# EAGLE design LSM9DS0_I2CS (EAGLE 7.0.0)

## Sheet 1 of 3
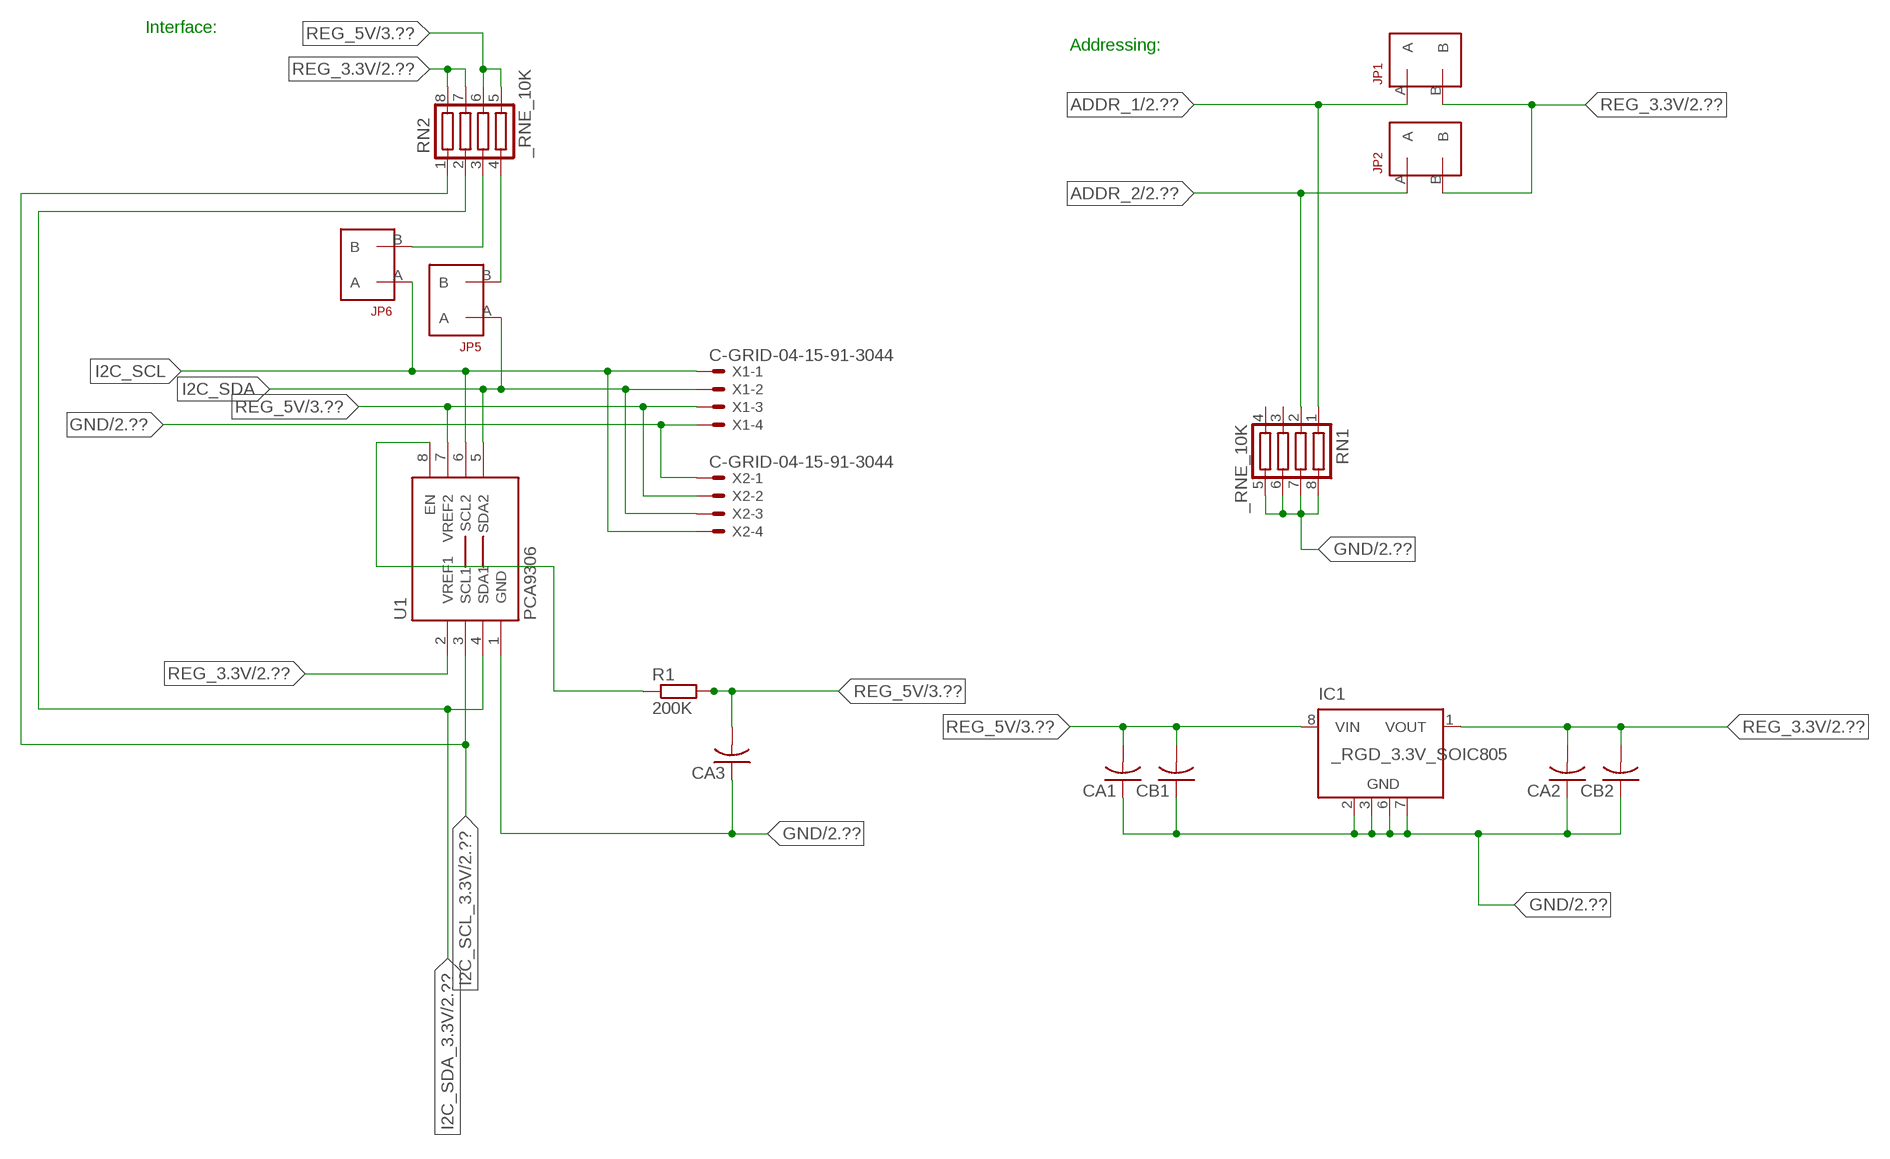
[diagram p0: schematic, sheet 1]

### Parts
CA1  CC1206KRX7R9BB104  [.1UF]
CA2  CC1206KRX7R9BB104  [.1UF]
CA3  CC1206KRX7R9BB104  [.1UF]
CB1  TMK316F106ZL-TC1206K  [TMK316F106ZL-T]
CB2  TMK316F106ZL-TC1206K  [TMK316F106ZL-T]
IC1  _RGD_3.3V_SOIC805  [_RGC_3.3V_SOIC8]
JP1  JUMPER_1X2_2MM  [JUMPER_1X2_2MM]
JP2  JUMPER_1X2_2MM  [JUMPER_1X2_2MM]
JP5  JUMPER_1X2_2MM  [JUMPER_1X2_2MM]
JP6  JUMPER_1X2_2MM  [JUMPER_1X2_2MM]
R1  200K  RESISTOR_SMT-0603  [R603]
RN1  _RNE_10K  [RNE]
RN2  _RNE_10K  [RNE]
U1  PCA9306  PCA9306_NCD  [PSOP-8]
X1  C-GRID-04-15-91-3044  [15-91-04]
X2  C-GRID-04-15-91-3044  [15-91-04]

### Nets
ADDR_1: JP1.A RN1.1 ; also sheet 2
ADDR_2: JP2.A RN1.2 ; also sheet 2
GND: CA1.1 CA2.1 CA3.1 CB1.1 CB2.1 IC1.2(GND) IC1.3(GND) IC1.6(GND) IC1.7(GND) RN1.5 RN1.6 RN1.7 RN1.8 U1.1(GND) X1.4 X2.1 ; also sheet 2,3
I2C_SCL: JP6.A U1.6(SCL2) X1.1 X2.4
I2C_SCL_3.3V: RN2.1 U1.3(SCL1) ; also sheet 2
I2C_SDA: JP5.A U1.5(SDA2) X1.2 X2.3
I2C_SDA_3.3V: RN2.2 U1.4(SDA1) ; also sheet 2
N$1: JP6.B RN2.3
N$2: JP5.B RN2.4
N$3: R1.1 U1.8(EN)
REG_3.3V: CA2.2 CB2.2 IC1.1(VOUT) JP1.B JP2.B RN2.7 RN2.8 U1.2(VREF1) ; also sheet 2
REG_5V: CA1.2 CA3.2 CB1.2 IC1.8(VIN) R1.2 RN2.5 RN2.6 U1.7(VREF2) X1.3 X2.2 ; also sheet 3
Unconnected: IC1.4(NC) IC1.5(NC) RN1.3 RN1.4

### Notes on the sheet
- Interface:
- Addressing:

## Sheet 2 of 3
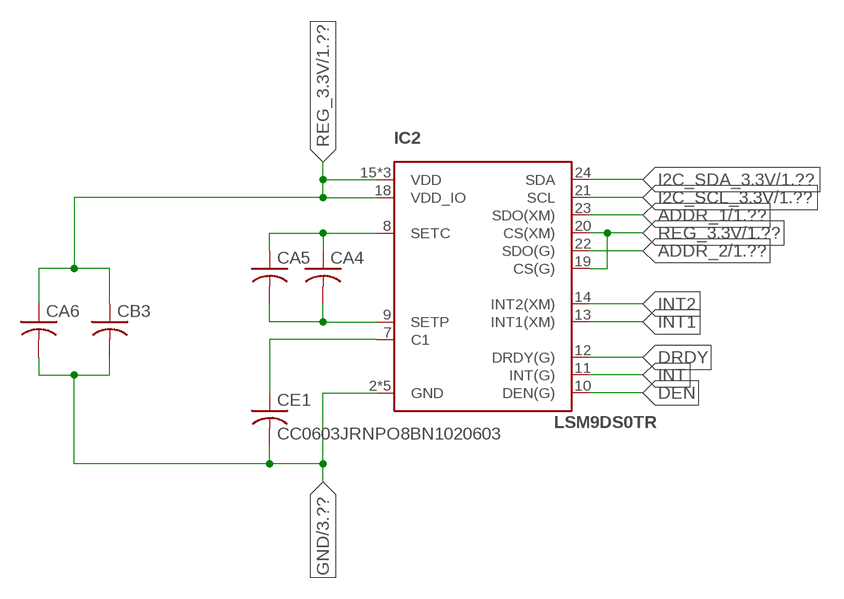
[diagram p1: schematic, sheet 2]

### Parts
CA4  CC1206KRX7R9BB104  [.1UF]
CA5  CC1206KRX7R9BB104  [.1UF]
CA6  CC1206KRX7R9BB104  [.1UF]
CB3  TMK316F106ZL-TC1206K  [TMK316F106ZL-T]
CE1  CC0603JRNPO8BN1020603  [CC0603JRNPO8BN102]
IC2  LSM9DS0TR  LSM9DS0  [LGA-24]

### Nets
ADDR_1: IC2.23(SDO(XM)) ; also sheet 1
ADDR_2: IC2.22(SDO(G)) ; also sheet 1
DEN: IC2.10(DEN(G))
DRDY: IC2.12(DRDY(G))
GND: CA6.2 CB3.2 CE1.2 IC2.2(GND) IC2.3(GND) IC2.4(GND) IC2.5(GND) IC2.6(GND) ; also sheet 1,3
I2C_SCL_3.3V: IC2.21(SCL) ; also sheet 1
I2C_SDA_3.3V: IC2.24(SDA) ; also sheet 1
INT: IC2.11(INT(G))
INT1: IC2.13(INT1(XM))
INT2: IC2.14(INT2(XM))
N$17: CA4.2 CA5.2 IC2.9(SETP)
N$18: CE1.1 IC2.7(C1)
N$19: CA4.1 CA5.1 IC2.8(SETC)
REG_3.3V: CA6.1 CB3.1 IC2.15(VDD) IC2.16(VDD) IC2.17(VDD) IC2.18(VDD_IO) IC2.19(CS(G)) IC2.20(CS(XM)) ; also sheet 1

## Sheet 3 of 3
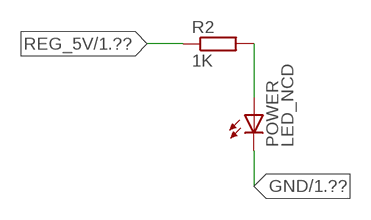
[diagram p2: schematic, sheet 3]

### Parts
POWER  LED_NCD  [CHIPLED_0603]
R2  1K  RESISTOR_SMT-0402  [R402]

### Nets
GND: POWER.C ; also sheet 1,2
N$4: POWER.A R2.2
REG_5V: R2.1 ; also sheet 1

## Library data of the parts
CA1-CA3 = NCD_ULTIMATE_LIBRARY:CC1206KRX7R9BB104: Capacitor CA .1uF 50V SMT C1206K CC1206KRX7R9BB104
CA4-CA6 = NCD_ULTIMATE_LIBRARY (2):CC1206KRX7R9BB104: Capacitor CA .1uF 50V SMT C1206K CC1206KRX7R9BB104
CB1 CB2 = NCD_ULTIMATE_LIBRARY:TMK316F106ZL-T: Capacitor CB 10uF SMT 1206 TMK316F106ZL-T
CB3 = NCD_ULTIMATE_LIBRARY (2):TMK316F106ZL-T: Capacitor CB 10uF SMT 1206 TMK316F106ZL-T
CE1 = NCD_ULTIMATE_LIBRARY (2):CC0603JRNPO8BN102: Capacitor CE 1uF SMT CC0603JRNPO8BN102 0603
IC1 = NCD_ULTIMATE_LIBRARY:_RGD_3.3V_SOIC8: Regulator Linear 3.3V Chip Positive VOLTAGE REGULATOR Digikey 497-1199-2-ND/L78L33ACD13TR
IC2 = NCD_ULTIMATE_KAMNA:LSM9DS0
JP1 JP2 JP5 JP6 = NCD_ULTIMATE_CONNECTORS:JUMPER_1X2_2MM
POWER = NCD_ULTIMATE_LIBRARY:LED_NCD: LED Digikey 754-1132-2-ND/APT2012SRCPRV
R1 R2 = NCD_ULTIMATE_LIBRARY:RESISTOR_SMT: NCD Resistor
RN1 RN2 = NCD_ULTIMATE_LIBRARY:_RNE_10K: Resistor Array RNE SMT 10K x 4 Single Resistor Source: http://www.ctscorp.com/components/Datasheets/CTSChipArrayDs.pdf Digikey 742C083103JPTR-ND/742C083103JP; OC_FARNELL: unknown; OC_NEWARK: unknown
U1 = NCD_ULTIMATE_LIBRARY:PCA9306_NCD: NCD Bidirectional I2C level shifter. NOT compatible with all available part number pinout schemes- DOUBLE CHECK!!!; PROD_ID: IC-10023
X1 X2 = NCD_ULTIMATE_CONNECTORS:C-GRID-04: CONNECTOR 4-Pos I2C wire to board 2.54 mm (0.100") pitch header Digikey WM1342-ND/0015912045; OC_FARNELL: unknown; OC_NEWARK: unknown

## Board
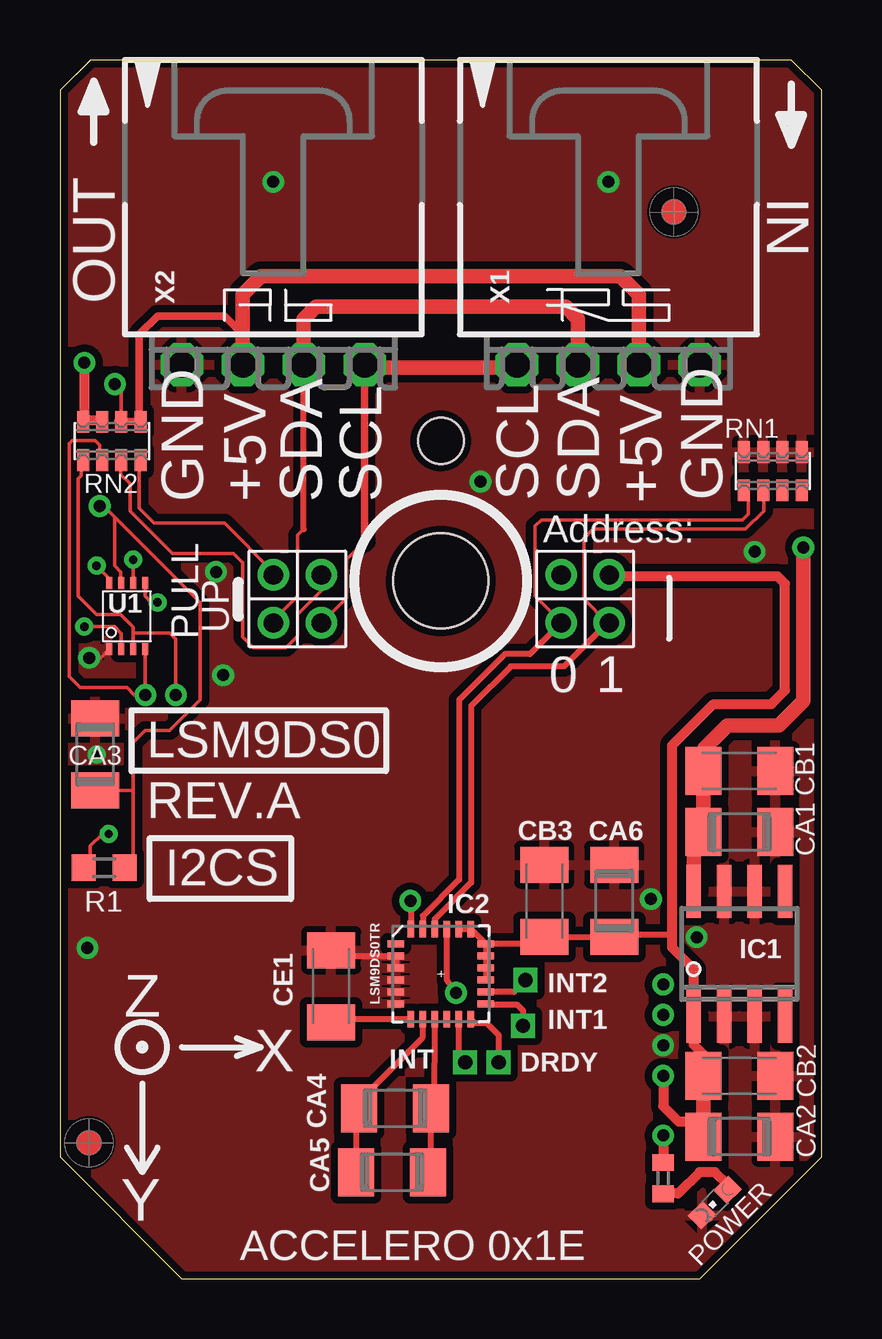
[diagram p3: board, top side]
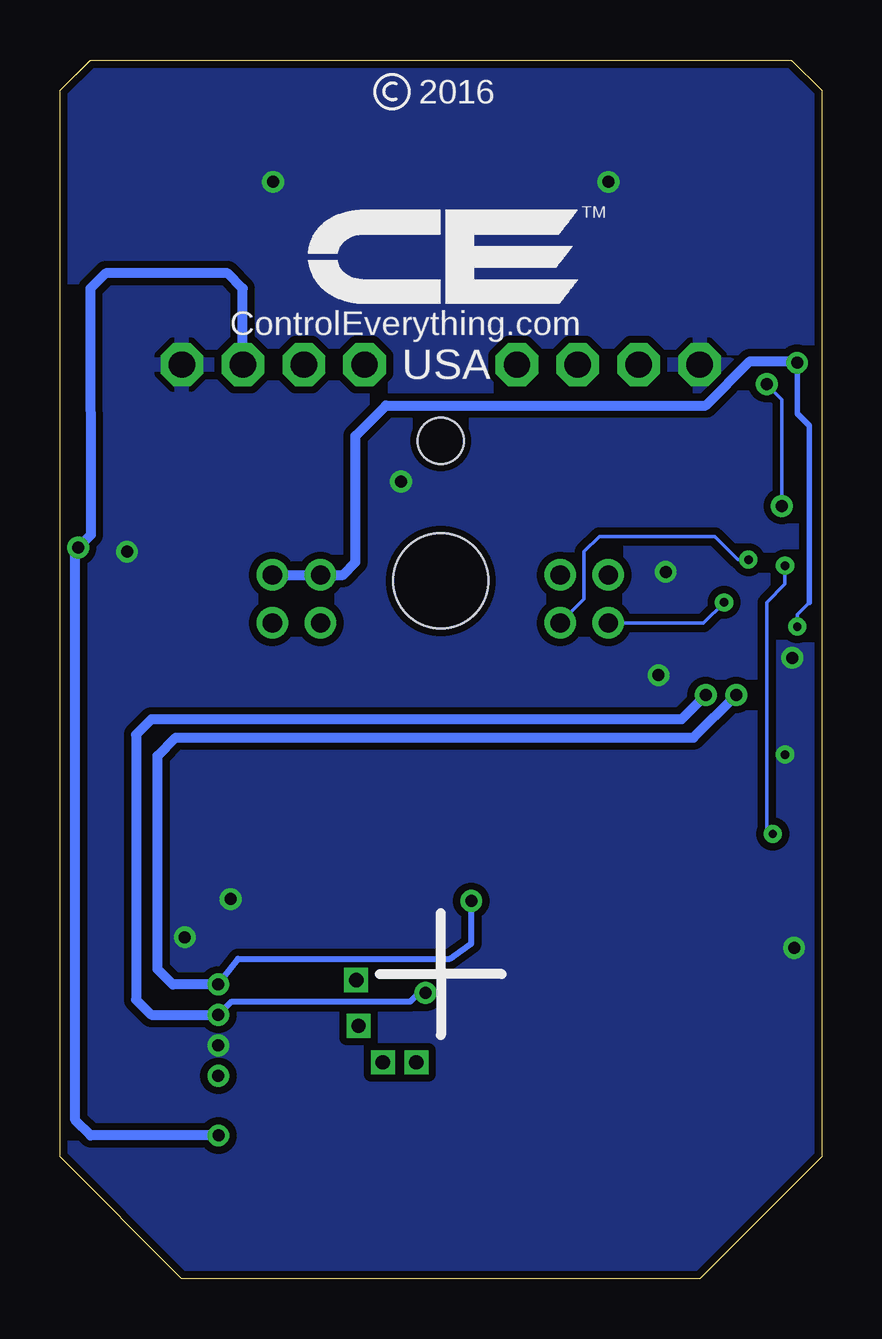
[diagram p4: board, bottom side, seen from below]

Size 31.75 x 50.8 mm. Coordinates in mm from the lower left corner, seen from the top.
Outline: 32 segments
Copper layers (1*16): Top 0.035mm / dielectric 1.5mm / Bottom 0.035mm
Design rules "default": minimum track width 5mil, minimum drill 24mil, track to track 5mil, track to pad 5mil, pad to pad 5mil, via to via 5mil, smd to smd 5mil, copper to edge 10mil, drill to drill 8mil, minimum pad ring 10mil, minimum via ring 8mil, stop-mask expansion 2mil, vias tented up to drill 0mil, thermal gap 10mil
Holes 3.96 mm at 15.88,29.08
Holes 1.91 mm at 15.88,34.93

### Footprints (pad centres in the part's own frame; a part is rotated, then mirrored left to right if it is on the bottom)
.1UF = smd 1.5 x 2: 1 -1.5,0; 2 1.5,0
TMK316F106ZL-T = smd 1.5 x 2: 1 -1.5,0; 2 1.5,0
CC0603JRNPO8BN102 = smd 1.5 x 2: 1 -1.5,0; 2 1.5,0
_RGC_3.3V_SOIC8 = smd 0.6 x 2.2: 1 -1.905,-2.6; 2 -0.635,-2.6; 3 0.635,-2.6; 4 1.905,-2.6; 5 1.905,2.6; 6 0.635,2.6; 7 -0.635,2.6; 8 -1.905,2.6
LGA-24 = smd 0.7 x 0.29: 1 -1.875,1.25; 2 -1.875,0.75; 3 -1.875,0.25; 4 -1.875,-0.25; 5 -1.875,-0.75; 6 -1.875,-1.25; 13 1.875,-1.25; 14 1.875,-0.75; 15 1.875,-0.25; 16 1.875,0.25; 17 1.875,0.75; 18 1.875,1.25 | smd 0.29 x 0.7: 7 -1.25,-1.875; 8 -0.75,-1.875; 9 -0.25,-1.875; 10 0.25,-1.875; 11 0.75,-1.875; 12 1.25,-1.875; 19 1.25,1.875; 20 0.75,1.875; 21 0.25,1.875; 22 -0.25,1.875; 23 -0.75,1.875; 24 -1.25,1.875
JUMPER_1X2_2MM = drill 0.8: A 0,2; B 0,0
CHIPLED_0603 = smd 0.8 x 0.876: A 0,-0.75; C 0,0.75
R603 = smd 1 x 1.1: 1 -0.85,0; 2 0.85,0
R402 = smd 0.7 x 0.9: 1 -0.65,0; 2 0.65,0
RNE = smd 0.5 x 0.9: 1 -1.2,-0.8; 2 -0.4,-0.8; 3 0.4,-0.8; 4 1.2,-0.8; 5 1.2,0.8; 6 0.4,0.8; 7 -0.4,0.8; 8 -1.2,0.8
PSOP-8 = smd 0.25 x 0.5: 1 -0.73,-1.37; 2 -0.23,-1.37; 3 0.27,-1.37; 4 0.77,-1.37; 5 0.77,1.38; 6 0.27,1.38; 7 -0.23,1.38; 8 -0.73,1.38
15-91-04 = drill 1.1 pad 1.778 octagon: 1 -3.81,-7.62; 2 -1.27,-7.62; 3 1.27,-7.62; 4 3.81,-7.62

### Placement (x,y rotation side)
CA1  28.32,18.62 180 top
CA2  28.32,5.92 180 top
CA3  1.46,21.86 270 top
CA4  13.97,7.11 0 top
CA5  13.84,4.45 0 top
CA6  23.11,15.75 90 top
CB1  28.32,21.16 180 top
CB2  28.32,8.46 180 top
CB3  20.19,15.75 90 top
CE1  11.3,12.19 90 top
IC1  28.32,13.54 0 top
IC2  15.88,12.7 0 top
JP1  20.89,29.34 180 top
JP2  22.9,29.34 180 top
JP5  8.89,29.34 180 top
JP6  10.9,29.34 180 top
POWER  27.3,3.18 135 top
R1  1.84,17.13 0 top
R2  25.15,4.19 270 top
RN1  29.72,33.66 0 top
RN2  2.16,34.93 0 top
U1  2.79,27.61 0 top
U$5  [VISION_REF10]  1.21,5.66 90 top
U$28  [VISION_REF10]  25.59,44.46 90 top
X1  22.86,45.72 0 top
X2  8.89,45.72 0 top

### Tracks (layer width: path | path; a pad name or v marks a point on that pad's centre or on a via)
ADDR_1
  Top 0.152: JP1.A 20.89,27.37 19.81,28.45 19.81,31.37 20.07,31.62 28.45,31.62 28.7,31.88 28.7,32.78 RN1.1
  Top 0.254: JP1.A 19.59,26.04 18.54,26.04 16.64,24.13 16.64,16.64 15.12,15.13 IC2.23
ADDR_2
  Top 0.152: JP2.A 22.83,27.34 21.84,28.32 21.84,30.86 22.23,31.24 28.57,31.24 29.34,32 29.34,32.59 RN1.2
  Top 0.254: 22.83,27.34 21.02,25.53 18.8,25.53 17.14,23.88 17.14,16.51 15.62,14.99 IC2.22
DRDY  (via drill 0.6)
  Top 0.254: IC2.12 17.28,10.67 17.78,10.67 18.29,10.16 v18.29,9.02
GND  (via drill 0.35, 0.5)
  Top 0.152: CA3.1 1.52,23.42 1.52,23.62 | U1.1 1.7,25.88 v1.22,25.88
  Top 0.254: CE1.2 11.54,13.45 IC2.2 IC2.3
  other vias: 8.89,45.72 22.86,45.72 25.15,9.73 6.8,25.16 17.53,33.22 26.55,14.24 1.15,13.79 6.5,29.46 1.52,21.84 24.64,15.82 28.96,30.3
  pour Top (isolate 0.305): -1.27,0 -1.27,50.8 33.02,50.8 33.02,0
  pour Bottom (isolate 0.305): -5.08,0 -5.08,50.8 35.56,50.8 35.56,0
I2C_SCL  (via drill 0.35)
  Top 0.152: 12.7,30.73 11.94,29.97 11.94,28.38 JP6.A | v3.05,29.97 3.06,29.96 U1.6
  Top 0.305: 12.7,30.73 X2.4
  Top 0.406: X2.4 12.7,37.97 | 19.05,37.97 X1.1
  Top 0.61: 12.7,37.97 19.05,37.97
  Bottom 0.152: JP6.A 9.91,28.33 9.91,30.3 9.27,30.94 4.45,30.94 3.48,29.97 v3.05,29.97
I2C_SCL_3.3V  (via drill 0.5)
  Top 0.152: RN2.1 0.89,34.07 0.89,33.48 0.77,33.35 0.77,29.1 0.76,29.09 0.76,28.45 1.52,27.69 2.54,27.69 3.06,27.17 3.06,26.92 | 3.06,26.92 U1.3 | v4.83,24.33 v4.83,24.34 4.83,26.67 4.57,26.92 3.06,26.92
  Top 0.254: v16.51,11.91 16.12,12.45 IC2.21
  Bottom 0.254: v25.15,11 24.59,11.56 17.14,11.56 16.89,11.81 v16.51,11.91
  Bottom 0.406: v4.83,24.33 5.84,23.32 27.94,23.32 28.58,22.68 28.58,11.63 27.94,11 v25.15,11
I2C_SDA  (via drill 0.35)
  Top 0.152: JP5.A 8.89,27.44 9.91,28.45 9.91,30.99 10.16,31.24 | U1.5 3.56,28.45 3.81,28.19 v4.06,28.19
  Top 0.254: 10.16,31.24 10.16,31.25 X2.3
  Top 0.61: X2.3 10.16,40.01 10.67,40.51 21.09,40.51 21.59,40.01 X1.2
  Bottom 0.152: v4.06,28.19 4.92,27.34 JP5.A
I2C_SDA_3.3V  (via drill 0.5)
  Top 0.152: RN2.2 1.65,34.14 1.65,34.75 1.46,34.94 0.51,34.94 0.38,34.81 0.38,26.37 0.38,26.36 0.38,25.1 0.84,24.64 2.79,24.64 3.1,24.33 v3.56,24.33 v3.56,24.34 U1.4
  Top 0.254: v14.61,15.75 14.62,15.73 IC2.24
  Bottom 0.254: 14.61,14.86 v14.61,15.75 14.61,13.97 15.49,13.34 24.34,13.34 v25.15,12.27
  Bottom 0.406: v25.15,12.27 27.05,12.27 27.69,12.9 27.69,21.79 26.93,22.56 5.34,22.56 v3.56,24.33
INT  (via drill 0.6)
  Top 0.254: v16.89,9.02 16.62,9.39 IC2.11
INT1  (via drill 0.6)
  Top 0.254: IC2.13 17.77,11.43 19.05,11.43 19.3,11.18 v19.3,10.54
INT2  (via drill 0.6)
  Top 0.254: v19.41,12.45 18.93,11.95 IC2.14
N$1
  Top 0.152: JP6.B 10.92,29.31 10.92,28.7 9.91,27.69 9.91,26.8 9.42,26.31 8.06,26.31 7.62,26.75 7.62,29.84 7.24,30.23 4.7,30.23 2.92,32 2.92,33.15 2.54,33.53 2.54,34.1 RN2.3
  Top 0.305: 2.54,34.02 RN2.3
N$2
  Top 0.152: JP5.B 8.89,29.46 6.86,31.5 3.94,31.5 3.3,32.13 3.3,34.07 RN2.4
  Top 0.305: 3.37,33.88 RN2.4
N$3  (via drill 0.35)
  Top 0.152: R1.1 1.27,17.41 1.27,18.03 1.78,18.54 v2.03,18.54 | v1.52,29.72 2.06,29.18 U1.8
  Bottom 0.152: v2.03,18.54 2.29,18.8 2.29,28.19 1.52,28.96 v1.52,29.72
N$4
  Top 0.406: POWER.A 27.84,3.92 27.3,4.45 26.67,4.45 25.78,3.56 25.16,3.56 R2.2
N$17
  Top 0.254: CA5.2 15.47,4.57 CA4.2 15.62,7.27 15.49,7.4 15.62,7.72 15.62,10.29 IC2.9
N$18
  Top 0.254: CE1.1 11.44,10.83 IC2.7
N$19
  Top 0.254: IC2.8 15.11,10.03 12.47,7.39 CA4.1 12.34,6.99 CA5.1
REG_3.3V  (via drill 0.35, 0.5)
  Top 0.152: v1.02,27.18 2.29,27.18 2.56,26.9 U1.2
  Top 0.254: IC2.18 IC2.17 IC2.16 IC2.15 | IC2.18 17.77,13.97 19.81,13.97 20.09,14.25 CB3.1 CA6.1 23.22,14.35 25.53,14.35 | IC2.20 IC2.19 IC2.18
  Top 0.406: CB2.2 26.82,9.35 26.42,9.75 26.42,10.36 | v25.15,8.46 25.15,7.19 25.78,6.55 26.82,6.55 | IC1.1 26.42,12.9 25.53,13.79 25.53,14.35 25.53,22.24 27.24,23.95 29.66,23.95 30.23,24.52 30.23,28.97 29.91,29.29 22.95,29.29 JP2.B | 26.52,5.62 CA2.2 | v1.02,38.18 1.02,35.78 | 1.02,35.78 RN2.8 | 1.02,35.78 1.71,35.78 RN2.7
  Top 0.61: CB2.2 26.82,6.55 CA2.2 | 26.42,10.36 IC1.1
  Bottom 0.152: 0.51,28.19 1.02,27.69 v1.02,27.18
  Bottom 0.229: 0.51,28.19 0.51,35.56 1.02,36.07 v1.02,38.18
  Bottom 0.406: v1.02,38.18 1.08,38.24 2.99,38.24 4.83,36.4 18.16,36.4 19.43,35.13 19.43,29.87 19.94,29.34 JP1.B JP2.B
REG_5V  (via drill 0.5)
  Top 0.152: RN2.6 2.56,37.01 v2.29,37.29 | R1.2 3.05,17.49 3.05,20.36 | 3.05,20.36 3.05,22.35 3.56,22.86 4.57,22.86 5.84,24.13 5.84,28.19 2.29,31.75 | CA3.2 3.05,20.36 | 2.29,31.75 1.83,32.21 v1.65,32.21 | U1.7 2.54,29.01 2.54,29.46 2.29,29.72 2.29,31.75
  Top 0.305: 7.62,39.37 7.5,39.37 | 2.42,35.74 RN2.6 RN2.5 3.31,35.8 3.31,39.37 4.07,40.13 6.86,40.13 7.62,39.37 | X2.2 7.62,39.37
  Top 0.406: v25.15,5.97 R2.1
  Top 0.61: X2.2 7.62,41.02 8.38,41.78 23.37,41.78 24.13,41.02 X1.3 | IC1.8 26.42,18.21 CA1.2 CB1.2 26.86,21.2 26.86,22.11 27.82,23.06 29.98,23.06 30.99,24.08 v30.99,30.48
  Bottom 0.152: v1.65,32.21 1.65,36.65 v2.29,37.29
  Bottom 0.406: X1.3 24.13,41.28 24.77,41.91 29.84,41.91 30.48,41.27 30.47,31 v30.99,30.48 31.11,30.36 31.11,6.6 30.48,5.97 v25.15,5.97

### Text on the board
tNames: IN | OUT | GND | +5V | SDA | SCL | SCL | SDA | +5V | GND | Address: | PULL | UP | 0 | 1 | LSM9DS0 | REV.A | I2CS | INT2 | Z | INT1 | X | INT | DRDY | Y | ACCELERO 0x1E
bNames: 2016 | TM | ControlEverything.com | USA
